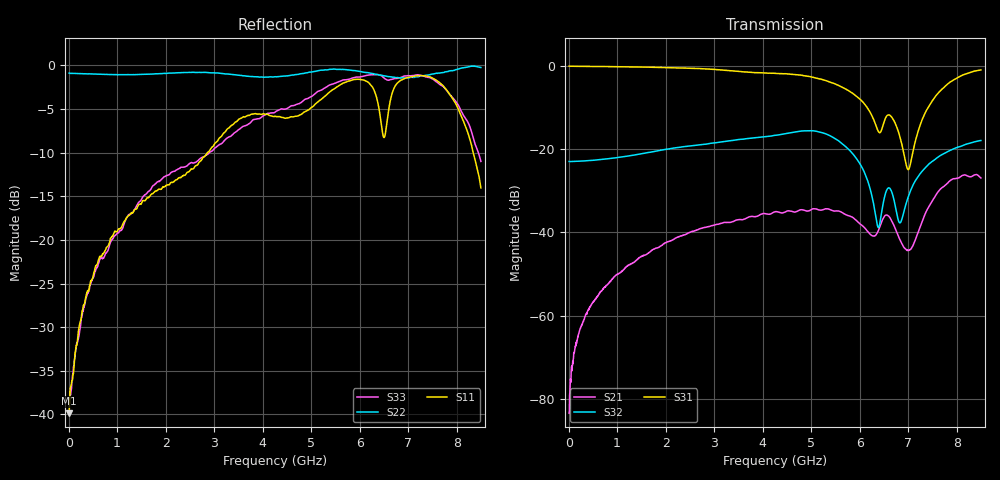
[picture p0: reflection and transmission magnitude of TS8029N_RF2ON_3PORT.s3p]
!Created with skrf (http://scikit-rf.org).
# GHz S RI R 50.0
!freq ReS11 ImS11 ReS12 ImS12 ReS13 ImS13
! ReS21 ImS21 ReS22 ImS22 ReS23 ImS23
! ReS31 ImS31 ReS32 ImS32 ReS33 ImS33
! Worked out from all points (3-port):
!   1601 points, 10 MHz to 8.5 GHz, reference 50 ohm
!   strongest paths, dB at 10 MHz, 2.132 GHz, 4.255 GHz, 6.378 GHz, 8.5 GHz:
!     S31: -0.1, -0.5, -1.9, -15.6, -1.0
!     S32: -23.0, -19.8, -16.7, -38.7, -18.0
!     S21: -83.3, -41.8, -35.1, -39.8, -26.9
!   lowest |S11| = -39.9 dB at 10 MHz (marker M1), VSWR 1.02, Z = 51 - j0.0199 ohm
!   |S11| at or under -10 dB: start of sweep to 2.862 GHz; 8.341 GHz to end of sweep
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0.01  0.0102 -0.000195  3.19e-05 2.37e-05  0.9845 -0.00471
      3.23e-05 5.99e-05  -0.9035 0.0034  0.071 -2.19e-06
      0.9845 -0.00487  0.071 4.92e-05  0.0115 -0.00242
0.2540875  0.00989 -0.0337  7.28e-05 0.000725  0.9752 -0.0905
           4.03e-05 0.000747  -0.8954 0.0608  0.0717 0.00073
           0.9758 -0.0906  0.0716 0.000743  0.00555 -0.0335
0.9598188  -0.0267 -0.1087  -0.000301 0.003  0.9139 -0.3279
           -0.000311 0.003  -0.8541 0.2392  0.0784 -0.0015
           0.9138 -0.3278  0.0784 -0.00162  -0.0234 -0.1039
4.255  -0.5105 0.0017  0.00828 0.0157  -0.0323 -0.8073
       0.00824 0.0156  -0.3343 0.7934  0.0687 -0.1285
       -0.0335 -0.8059  0.0685 -0.1288  -0.537 -0.0523
6.006062  -0.3496 0.7549  0.0107 0.00693  -0.3162 -0.2396
          0.0107 0.00692  -0.0367 0.9237  -0.0594 -0.0298
          -0.3162 -0.2393  -0.0596 -0.0297  -0.601 0.6138
6.382806  -0.011 0.5979  0.00376 0.00974  -0.1176 -0.1139
          0.00372 0.00972  0.0143 0.8845  -0.00552 -0.0101
          -0.1176 -0.1141  -0.00547 -0.0101  -0.3886 0.7957
6.658731  -0.4124 0.5342  0.0107 0.00884  -0.1559 -0.1852
          0.0107 0.00881  0.0953 0.8543  -0.00917 -0.0296
          -0.1564 -0.1849  -0.00911 -0.0296  -0.1235 0.8237
7.003637  -0.1125 0.8469  0.00169 0.00588  -0.000331 -0.0566
          0.00168 0.00591  0.2465 0.8139  0.0213 -0.0164
          -0.000341 -0.0567  0.0213 -0.0164  0.253 0.8362
7.741206  0.5681 0.4968  -0.00483 0.0355  0.2861 -0.4678
          -0.00481 0.0355  0.5046 0.7604  0.0445 -0.0763
          0.2853 -0.4683  0.0444 -0.0762  0.5641 0.4914
8.5  0.1782 0.0882  0.0191 0.0408  -0.1043 -0.8816
     0.0191 0.0408  0.4693 0.8528  0.0313 -0.1227
     -0.1054 -0.8817  0.0313 -0.1227  0.2778 0.0486
